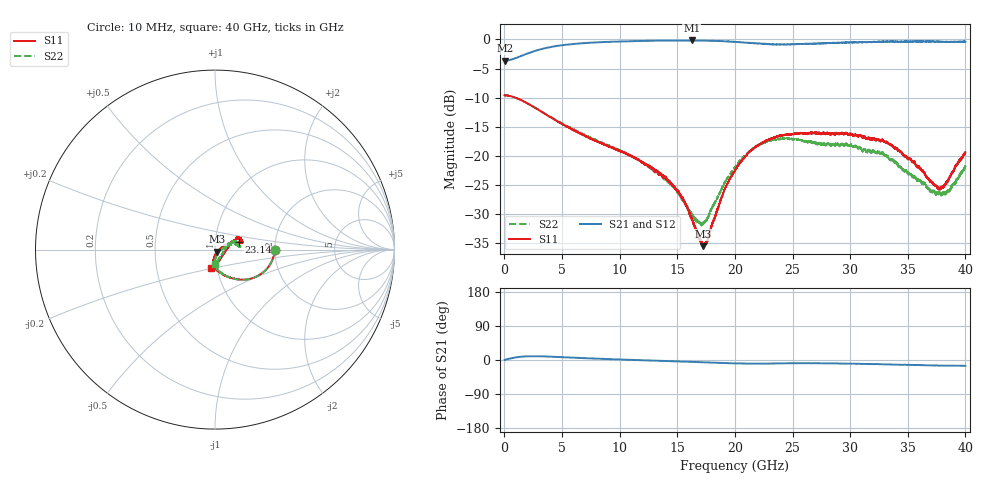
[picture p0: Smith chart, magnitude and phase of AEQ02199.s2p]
! Sonnet Data File
! From: emgraph Version : 16.52
! From Emgraph Data: 2
! Data File Written: 02/28/2018 11:08:11
!< HDATE 02/28/2018 11:04:21
!< MDATE 02/28/2018 11:04:21
# GHZ S MA R 50.00000
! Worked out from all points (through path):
!   12801 points, 10 MHz to 40 GHz, reference 50 ohm
!   highest |S21| = -0.18 dB at 16.26 GHz (marker M1); lowest = -3.7 dB at 19.37 MHz (marker M2)
!   group delay of S21, straight-line fit = 1.7 ps
!   lowest |S11| = -35.5 dB at 17.24 GHz (marker M3), VSWR 1.03, Z = 51.2 - j1.18 ohm
!   |S11| at or under -10 dB: 960.5 MHz to end of sweep
!   |S22| runs from -31.9 to -9.6 dB; largest |S21 - S12| = 0.03
!   S11 on the Smith chart (normalised r, x): 10 MHz: 1.99, -0.01; 23.14 GHz: 1.31, +0.11; 40 GHz: 0.93, -0.20
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0.01  0.3321 -0.3  0.659 0.1  0.6578 0.1  0.3328 -0.0
0.01937266  0.3312 -0.4  0.6561 0.2  0.6577 0.2  0.3306 -0.4
1.262812  0.3074 -20.8  0.7089 8.0  0.7097 8.0  0.3071 -20.8
2.46876  0.2655 -36.2  0.7865 10.0  0.7869 10.0  0.2661 -36.2
6.677083  0.154 -69.0  0.9253 5.2  0.928 5.0  0.1567 -67.9
10.75731  0.1024 -89.7  0.9642 0.6  0.9701 0.5  0.1028 -85.5
13.34104  0.07334 -97.1  0.9752 -2.0  0.9708 -2.7  0.07204 -89.8
15.11872  0.04964 -95.2  0.9787 -3.8  0.9823 -3.9  0.04799 -85.5
16.25594  0.02894 -86.3  0.9794 -4.9  0.9756 -5.0  0.03189 -66.1
17.24319  0.01684 -43.2  0.9759 -6.0  0.9757 -6.2  0.02624 -28.4
17.57748  0.01866 -17.3  0.975 -6.4  0.9747 -6.5  0.02865 -13.7
19.03337  0.04929 22.3  0.9639 -8.0  0.9645 -8.1  0.05709 15.0
20.005  0.07548 24.5  0.95 -8.9  0.9515 -8.7  0.07986 17.3
21.27656  0.1089 21.8  0.9328 -9.4  0.935 -9.5  0.1099 15.8
23.14172  0.1405 16.7  0.9068 -9.4  0.9031 -8.6  0.1362 9.5
26.67208  0.1572 16.1  0.9178 -8.7  0.9083 -7.8  0.1314 9.3
29.77131  0.1531 23.9  0.94 -9.7  0.9318 -9.4  0.1233 19.5
33.33604  0.127 25.6  0.9577 -11.8  0.9633 -11.4  0.09605 21.2
35.45739  0.08792 20.6  0.9558 -12.9  0.9574 -12.6  0.06579 21.2
37.74431  0.05292 -33.2  0.9542 -14.6  0.9524 -14.2  0.04624 -28.8
38.51912  0.06228 -65.3  0.9521 -14.9  0.9501 -14.2  0.04934 -55.4
40  0.1073 -103.0  0.9566 -15.4  0.9507 -14.0  0.0805 -88.7
